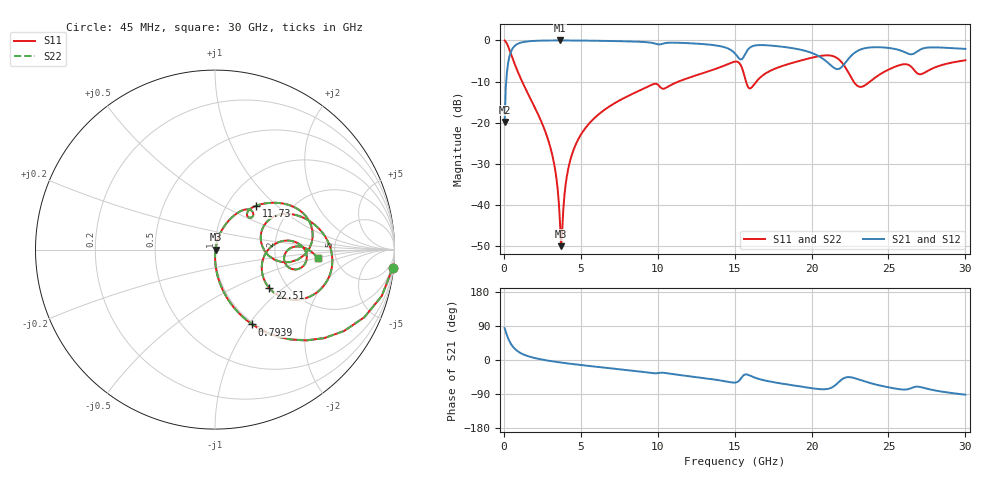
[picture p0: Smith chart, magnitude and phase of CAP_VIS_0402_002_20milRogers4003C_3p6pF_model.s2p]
! S-parameter model data by Modelithics Inc.  support@modelithics.com  813-866-6335  Tampa FL USA
! S-Parameter data specifications:
! Substrate: 20-mil Rogers 4003C, substrate thickness, H=0.508mm, Dielectric constant, Er=3.75
! PCB Mounting Pad Footprint: Pad width, PadW=0.50mm , Pad length, PadL=0.50mm , Pad gap, PadG (edge-to-edge)=0.40mm , Reference planes=1.4mm apart
! Created Wed Nov 18 12:46:53 2015
# hz S ma R 50
! 2 Port Network Data from SP1.SP block
! freq  magS11  angS11  magS21  angS21  magS12  angS12  magS22  angS22
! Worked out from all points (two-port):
!   401 points, 45 MHz to 30 GHz, reference 50 ohm
!   highest |S21| = -0.03 dB at 3.64 GHz (marker M1); lowest = -19.8 dB at 45 MHz (marker M2)
!   |S21| within 3 dB of the highest: 433.1 MHz to 14.98 GHz (14.55 GHz wide, 189 % of centre); 15.73 GHz to 19.99 GHz (4.268 GHz wide, 23.9 % of centre)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
!   lowest |S11| = -50.0 dB at 3.714 GHz (marker M3), VSWR 1.01, Z = 50.3 - j0.123 ohm
!   |S11| at or under -10 dB: 1.182 GHz to 11.35 GHz (10.17 GHz wide, 162 % of centre); 15.74 GHz to 16.41 GHz (673.3 MHz wide, 4.19 % of centre); 22.73 GHz to 23.8 GHz (1.065 GHz wide, 4.58 % of centre)
!   |S22| runs from -50.0 to 0.0 dB; largest |S21 - S12| = 0
!   S11 on the Smith chart (normalised r, x): 45 MHz: 1, -19; 793.9 MHz: 0.98, -1.04; 11.73 GHz: 1.36, +0.75; 22.51 GHz: 1.62, -0.81; 30 GHz: 3.61, -0.50
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4.5e7  0.9948 -5.9  0.1021 84.1  0.1021 84.1  0.9948 -5.9
3.4455e8  0.7833 -39.0  0.621 50.9  0.621 50.9  0.7833 -39.0
7.93875e8  0.466 -63.5  0.8835 26.3  0.8835 26.3  0.466 -63.5
2.965612e9  0.05457 -89.5  0.9957 -2.3  0.9957 -2.3  0.05457 -89.5
3.34005e9  0.02625 -88.3  0.9967 -4.6  0.9967 -4.6  0.02625 -88.3
3.6396e9  0.006456 -68.4  0.9968 -6.3  0.9968 -6.3  0.006456 -68.4
3.714488e9  0.003177 -22.6  0.9968 -6.8  0.9968 -6.8  0.003177 -22.6
4.2387e9  0.03086 74.4  0.9961 -9.5  0.9961 -9.5  0.03086 74.4
5.062462e9  0.07457 73.7  0.9934 -13.5  0.9934 -13.5  0.07457 73.7
1.007992e10  0.2819 41.4  0.8921 -34.3  0.8921 -34.3  0.2819 41.4
1.172745e10  0.3363 46.7  0.9288 -41.1  0.9288 -41.1  0.3363 46.7
1.50225e10  0.552 14.1  0.6921 -59.6  0.6921 -59.6  0.552 14.1
1.554671e10  0.424 -9.5  0.6145 -41.5  0.6145 -41.5  0.424 -9.5
1.599604e10  0.2603 10.5  0.8171 -41.2  0.8171 -41.2  0.2603 10.5
1.74189e10  0.436 27.2  0.8618 -57.8  0.8618 -57.8  0.436 27.2
2.003996e10  0.617 6.9  0.7005 -74.6  0.7005 -74.6  0.617 6.9
2.131305e10  0.6495 -15.1  0.4868 -72.6  0.4868 -72.6  0.6495 -15.1
2.251125e10  0.3716 -35.4  0.6312 -45.4  0.6312 -45.4  0.3716 -35.4
2.326012e10  0.2735 -10.4  0.7832 -54.0  0.7832 -54.0  0.2735 -10.4
2.505742e10  0.4462 5.6  0.8069 -72.5  0.8069 -72.5  0.4462 5.6
2.655518e10  0.4619 -13.9  0.6797 -73.0  0.6797 -73.0  0.4619 -13.9
3e10  0.5736 -4.7  0.7872 -91.6  0.7872 -91.6  0.5736 -4.7
